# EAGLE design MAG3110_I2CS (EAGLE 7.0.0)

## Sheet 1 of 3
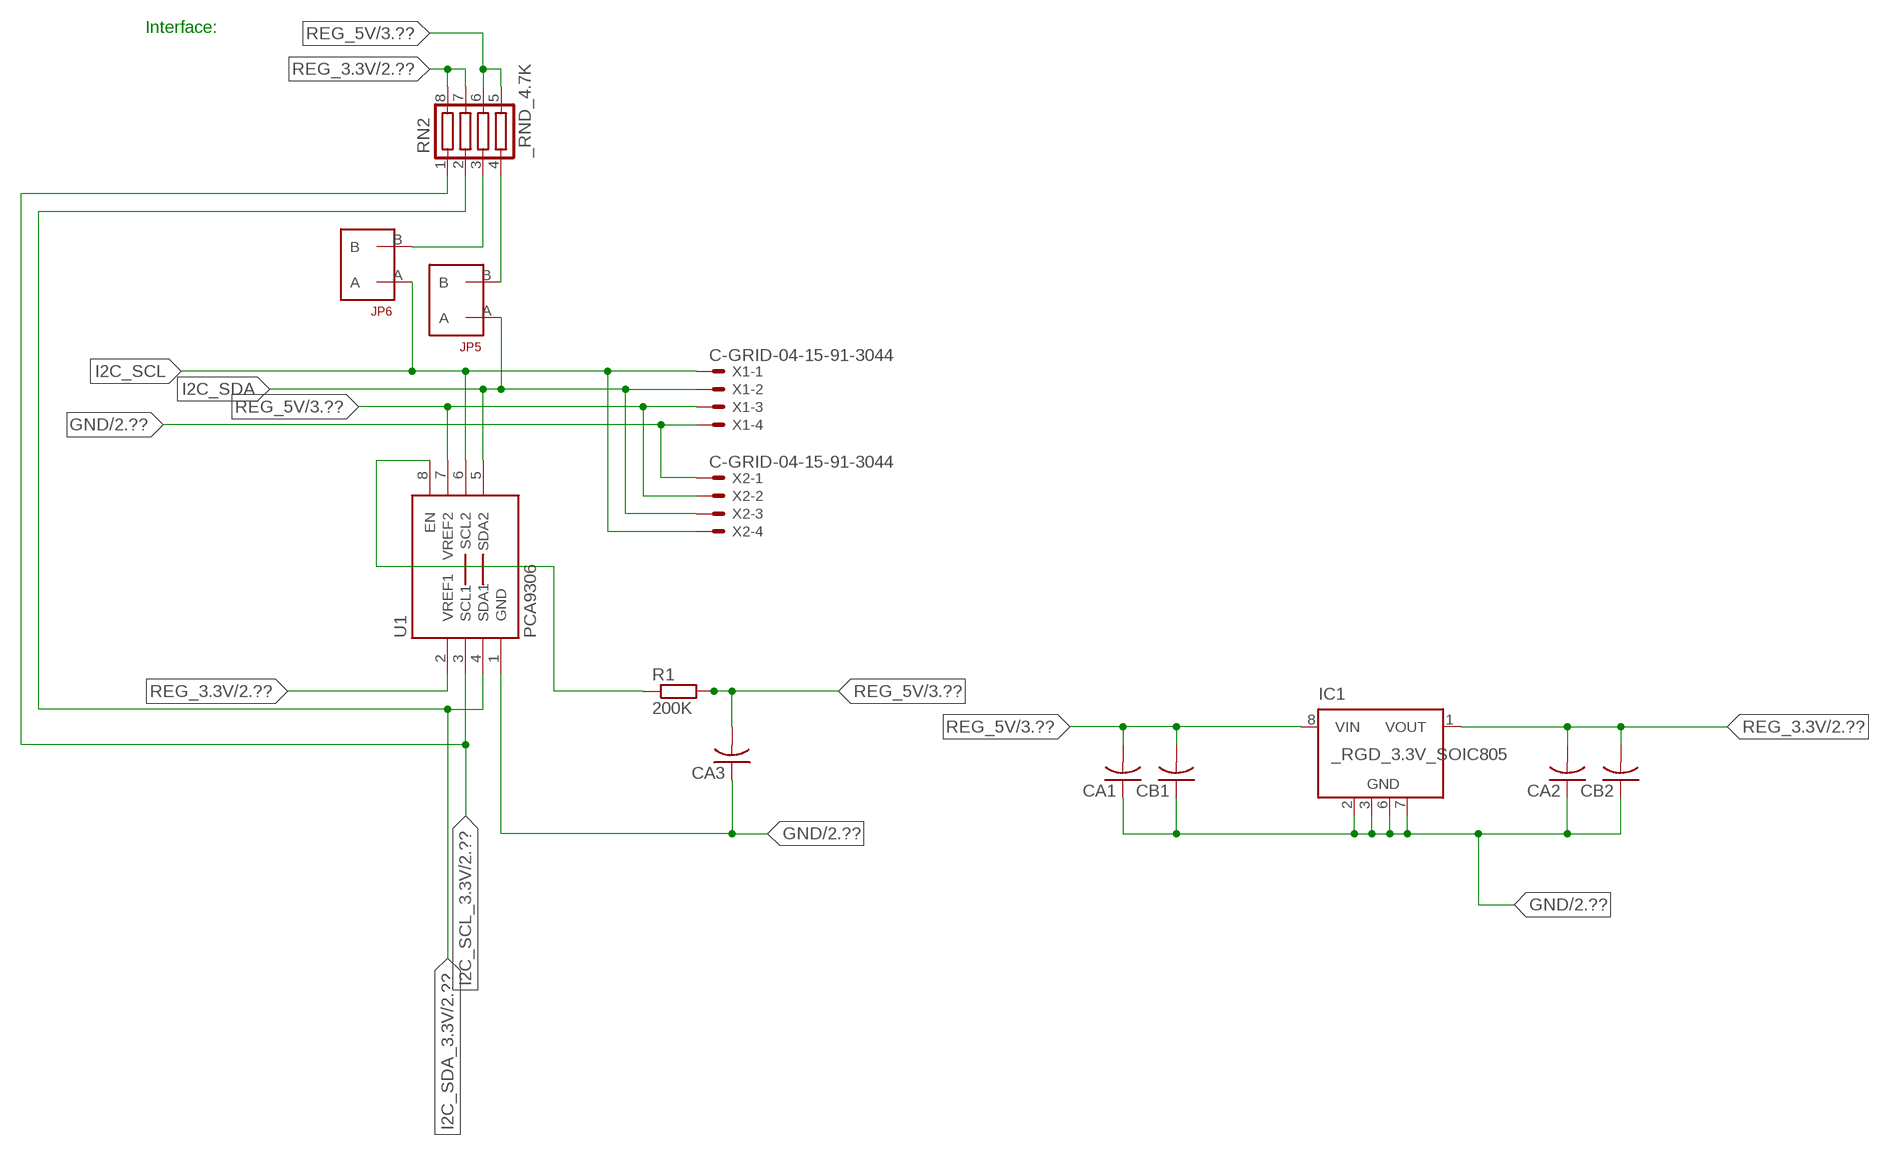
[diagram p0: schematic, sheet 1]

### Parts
CA1  CC1206KRX7R9BB104  [.1UF]
CA2  CC1206KRX7R9BB104  [.1UF]
CA3  CC1206KRX7R9BB104  [.1UF]
CB1  TMK316F106ZL-TC1206K  [TMK316F106ZL-T]
CB2  TMK316F106ZL-TC1206K  [TMK316F106ZL-T]
IC1  _RGD_3.3V_SOIC805  [_RGC_3.3V_SOIC8]
JP5  JUMPER_1X2_2MM  [JUMPER_1X2_2MM]
JP6  JUMPER_1X2_2MM  [JUMPER_1X2_2MM]
R1  200K  RESISTOR_SMT-0603  [R603]
RN2  _RND_4.7K  [RND]
U1  PCA9306  PCA9306_NCD  [PSOP-8]
X1  C-GRID-04-15-91-3044  [15-91-04]
X2  C-GRID-04-15-91-3044  [15-91-04]

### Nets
GND: CA1.1 CA2.1 CA3.1 CB1.1 CB2.1 IC1.2(GND) IC1.3(GND) IC1.6(GND) IC1.7(GND) U1.1(GND) X1.4 X2.1 ; also sheet 2,3
I2C_SCL: JP6.A U1.6(SCL2) X1.1 X2.4
I2C_SCL_3.3V: RN2.1 U1.3(SCL1) ; also sheet 2
I2C_SDA: JP5.A U1.5(SDA2) X1.2 X2.3
I2C_SDA_3.3V: RN2.2 U1.4(SDA1) ; also sheet 2
N$1: JP6.B RN2.3
N$2: JP5.B RN2.4
N$3: R1.1 U1.8(EN)
REG_3.3V: CA2.2 CB2.2 IC1.1(VOUT) RN2.7 RN2.8 U1.2(VREF1) ; also sheet 2
REG_5V: CA1.2 CA3.2 CB1.2 IC1.8(VIN) R1.2 RN2.5 RN2.6 U1.7(VREF2) X1.3 X2.2 ; also sheet 3
Unconnected: IC1.4(NC) IC1.5(NC)

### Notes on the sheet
- Interface:

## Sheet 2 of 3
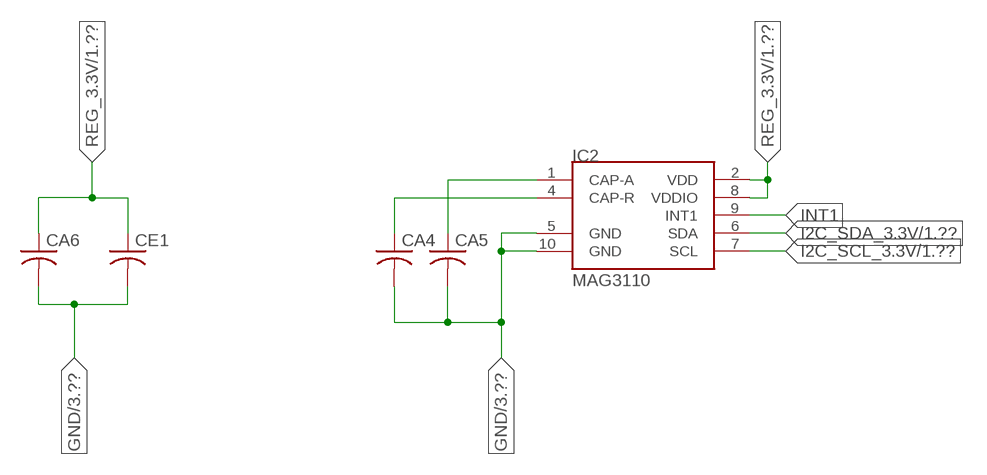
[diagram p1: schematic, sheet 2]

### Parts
CA4  CC1206KRX7R9BB104  [.1UF]
CA5  CC1206KRX7R9BB104  [.1UF]
CA6  CC1206KRX7R9BB104  [.1UF]
CE1  CC0603JRNPO8BN1020603  [CC0603JRNPO8BN102]
IC2  MAG3110  [DFN-10]

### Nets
GND: CA4.2 CA5.2 CA6.2 CE1.2 IC2.5(GND) IC2.10(GND) ; also sheet 1,3
I2C_SCL_3.3V: IC2.7(SCL) ; also sheet 1
I2C_SDA_3.3V: IC2.6(SDA) ; also sheet 1
INT1: IC2.9(INT1)
N$5: CA5.1 IC2.1(CAP-A)
N$6: CA4.1 IC2.4(CAP-R)
REG_3.3V: CA6.1 CE1.1 IC2.2(VDD) IC2.8(VDDIO) ; also sheet 1

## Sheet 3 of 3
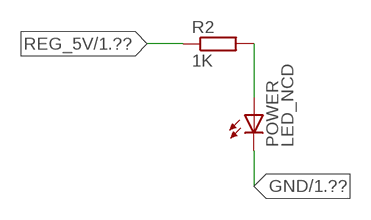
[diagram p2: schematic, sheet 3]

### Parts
POWER  LED_NCD  [CHIPLED_0603]
R2  1K  RESISTOR_SMT-0402  [R402]

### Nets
GND: POWER.C ; also sheet 1,2
N$4: POWER.A R2.2
REG_5V: R2.1 ; also sheet 1

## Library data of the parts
CA1-CA6 = NCD_ULTIMATE_LIBRARY:CC1206KRX7R9BB104: Capacitor CA .1uF 50V SMT C1206K CC1206KRX7R9BB104
CB1 CB2 = NCD_ULTIMATE_LIBRARY:TMK316F106ZL-T: Capacitor CB 10uF SMT 1206 TMK316F106ZL-T
CE1 = NCD_ULTIMATE_LIBRARY:CC0603JRNPO8BN102: Capacitor CE 1uF SMT CC0603JRNPO8BN102 0603
IC1 = NCD_ULTIMATE_LIBRARY:_RGD_3.3V_SOIC8: Regulator Linear 3.3V Chip Positive VOLTAGE REGULATOR Digikey 497-1199-2-ND/L78L33ACD13TR
IC2 = SparkFun-Sensors:MAG3110: 3-axis digital (I2C) magnetometer
JP5 JP6 = NCD_ULTIMATE_CONNECTORS:JUMPER_1X2_2MM
POWER = NCD_ULTIMATE_LIBRARY:LED_NCD: LED Digikey 754-1132-2-ND/APT2012SRCPRV
R1 R2 = NCD_ULTIMATE_LIBRARY:RESISTOR_SMT: NCD Resistor
RN2 = NCD_ULTIMATE_LIBRARY:_RND_4.7K: Resistor Array RND SMT 4.7K x 4 Single Resistor Source: http://www.ctscorp.com/components/Datasheets/CTSChipArrayDs.pdf Digikey 742C083472JPTR-ND/742C083472JP; OC_FARNELL: unknown; OC_NEWARK: unknown
U1 = NCD_ULTIMATE_LIBRARY:PCA9306_NCD: NCD Bidirectional I2C level shifter. NOT compatible with all available part number pinout schemes- DOUBLE CHECK!!!; PROD_ID: IC-10023
X1 X2 = NCD_ULTIMATE_CONNECTORS:C-GRID-04: CONNECTOR 4-Pos I2C wire to board 2.54 mm (0.100") pitch header Digikey WM1342-ND/0015912045; OC_FARNELL: unknown; OC_NEWARK: unknown

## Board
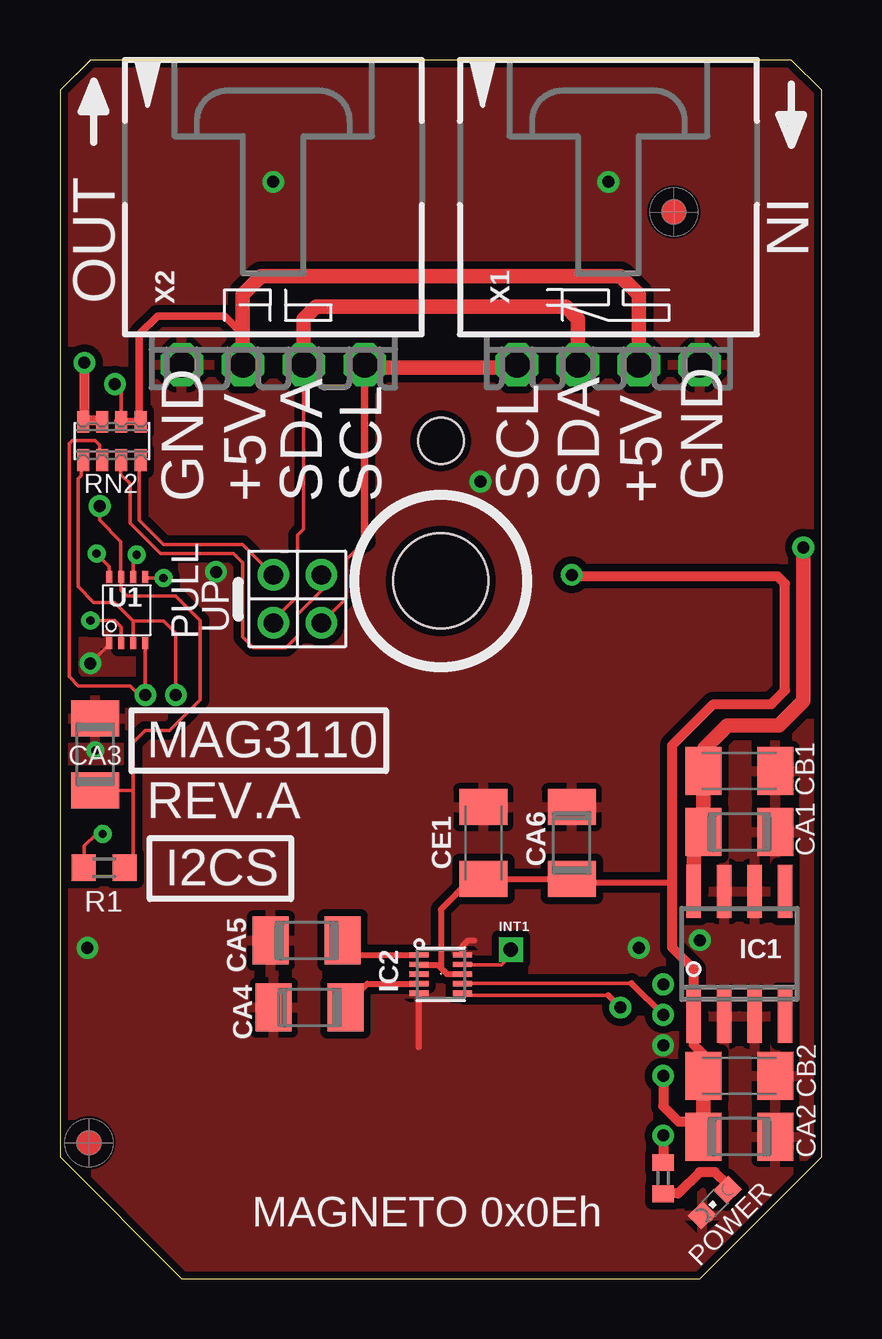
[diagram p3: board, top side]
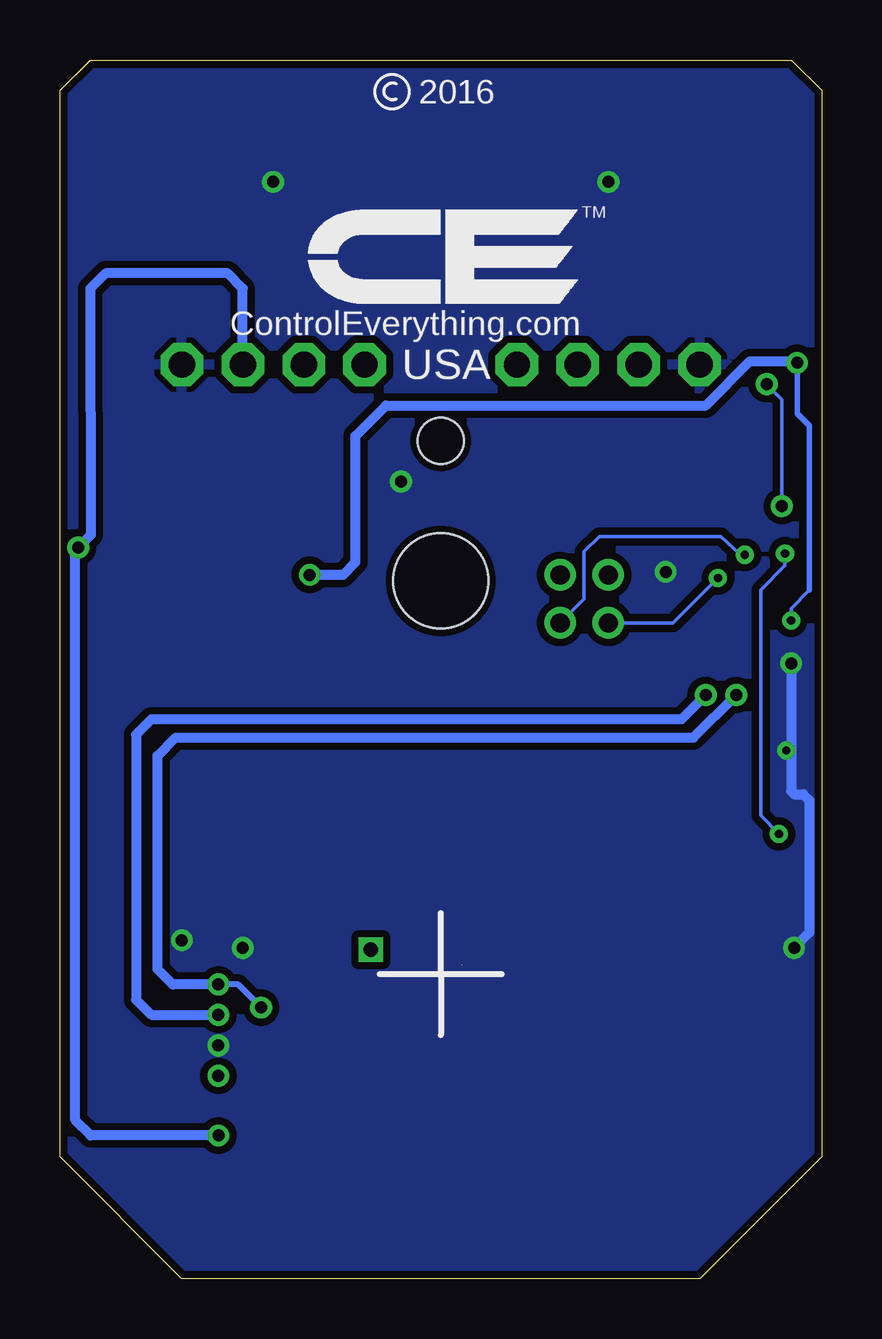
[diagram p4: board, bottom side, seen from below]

Size 31.75 x 50.8 mm. Coordinates in mm from the lower left corner, seen from the top.
Outline: 32 segments
Copper layers (1*16): Top 0.035mm / dielectric 1.5mm / Bottom 0.035mm
Design rules "default": minimum track width 5mil, minimum drill 24mil, track to track 5mil, track to pad 5mil, pad to pad 5mil, via to via 5mil, smd to smd 5mil, copper to edge 10mil, drill to drill 8mil, minimum pad ring 10mil, minimum via ring 8mil, stop-mask expansion 2mil, vias tented up to drill 0mil, thermal gap 10mil
Holes 3.96 mm at 15.88,29.08
Holes 1.91 mm at 15.88,34.93

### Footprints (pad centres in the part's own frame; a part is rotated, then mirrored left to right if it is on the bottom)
.1UF = smd 1.5 x 2: 1 -1.5,0; 2 1.5,0
TMK316F106ZL-T = smd 1.5 x 2: 1 -1.5,0; 2 1.5,0
CC0603JRNPO8BN102 = smd 1.5 x 2: 1 -1.5,0; 2 1.5,0
_RGC_3.3V_SOIC8 = smd 0.6 x 2.2: 1 -1.905,-2.6; 2 -0.635,-2.6; 3 0.635,-2.6; 4 1.905,-2.6; 5 1.905,2.6; 6 0.635,2.6; 7 -0.635,2.6; 8 -1.905,2.6
DFN-10 = smd 0.8 x 0.22: 1 -0.91,0.8; 2 -0.91,0.4; 3 -0.91,0; 4 -0.91,-0.4; 5 -0.91,-0.8; 6 0.91,-0.8; 7 0.91,-0.4; 8 0.91,0; 9 0.91,0.4; 10 0.91,0.8
JUMPER_1X2_2MM = drill 0.8: A 0,2; B 0,0
CHIPLED_0603 = smd 0.8 x 0.876: A 0,-0.75; C 0,0.75
R603 = smd 1 x 1.1: 1 -0.85,0; 2 0.85,0
R402 = smd 0.7 x 0.9: 1 -0.65,0; 2 0.65,0
RND = smd 0.5 x 0.9: 1 -1.2,-0.8; 2 -0.4,-0.8; 3 0.4,-0.8; 4 1.2,-0.8; 5 1.2,0.8; 6 0.4,0.8; 7 -0.4,0.8; 8 -1.2,0.8
PSOP-8 = smd 0.25 x 0.5: 1 -0.73,-1.37; 2 -0.23,-1.37; 3 0.27,-1.37; 4 0.77,-1.37; 5 0.77,1.38; 6 0.27,1.38; 7 -0.23,1.38; 8 -0.73,1.38
15-91-04 = drill 1.1 pad 1.778 octagon: 1 -3.81,-7.62; 2 -1.27,-7.62; 3 1.27,-7.62; 4 3.81,-7.62

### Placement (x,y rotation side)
CA1  28.32,18.62 180 top
CA2  28.32,5.92 180 top
CA3  1.46,21.86 270 top
CA4  10.41,11.3 180 top
CA5  10.29,14.1 180 top
CA6  21.34,18.16 90 top
CB1  28.32,21.16 180 top
CB2  28.32,8.46 180 top
CE1  17.65,18.16 90 top
IC1  28.32,13.54 0 top
IC2  15.88,12.7 0 top
JP5  8.89,29.34 180 top
JP6  10.9,29.34 180 top
POWER  27.3,3.18 135 top
R1  1.84,17.13 0 top
R2  25.15,4.19 270 top
RN2  2.16,34.93 0 top
U1  2.79,27.86 0 top
U$5  [VISION_REF10]  1.21,5.66 90 top
U$28  [VISION_REF10]  25.59,44.46 90 top
X1  22.86,45.72 0 top
X2  8.89,45.72 0 top

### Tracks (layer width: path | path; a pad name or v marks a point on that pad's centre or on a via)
GND  (via drill 0.35, 0.5)
  Top 0.152: CA3.1 1.52,23.42 1.52,23.62 | v1.27,25.65 2.06,26.45 U1.1
  Top 0.254: 14.96,9.65 IC2.5 | IC2.10 16.79,13.86 17.02,14.1 17.27,14.1
  Bottom 0.152: 1.27,20.32 1.14,20.19
  Bottom 0.406: v1.15,13.79 0.51,14.43 0.51,19.94 0.76,20.19 1.14,20.19 | v1.27,25.65 1.27,20.32
  other vias: 8.89,45.72 22.86,45.72 25.15,9.73 17.53,33.22 26.67,14.11 6.5,29.46 1.47,22.02 24.13,13.79
  pour Bottom (isolate 0.305): -0.64,5.08 -0.64,49.53 1.27,51.44 30.48,51.44 32.38,49.53 32.38,5.08 26.67,-0.63 5.08,-0.63
  pour Top (isolate 0.305): 4.45,-1.27 -1.27,4.45 -1.27,50.17 0.64,52.07 31.11,52.07 33.02,50.17 33.02,4.45 27.3,-1.27
I2C_SCL  (via drill 0.35)
  Top 0.152: 12.7,30.73 11.94,29.97 11.94,28.38 JP6.A | v3.2,30.18 3.06,29.99 U1.6
  Top 0.305: 12.7,30.73 X2.4
  Top 0.406: X2.4 12.7,37.97 | 19.05,37.97 X1.1
  Top 0.61: 12.7,37.97 19.05,37.97
  Bottom 0.152: JP6.A 9.91,28.33 9.91,30.3 9.27,30.94 4.19,30.94 3.38,30.18 v3.2,30.18
I2C_SCL_3.3V  (via drill 0.5)
  Top 0.152: RN2.1 0.89,34.07 0.89,33.48 0.77,33.35 0.77,28.84 1.41,28.19 2.29,28.19 3.06,27.42 | 23.83,12.32 16.8,12.32 IC2.7 | 3.06,27.42 U1.3 | v4.83,24.33 v4.83,24.34 4.83,26.92 4.33,27.42 3.06,27.42
  Top 0.254: 23.83,12.32 v25.15,11
  Bottom 0.406: v4.83,24.33 5.84,23.32 27.94,23.32 28.58,22.68 28.58,11.63 27.94,11 v25.15,11
I2C_SDA  (via drill 0.35)
  Top 0.152: JP5.A 8.89,27.44 9.91,28.45 9.91,30.99 10.16,31.24 10.16,34.92 X2.3 | U1.5 3.6,29.21 v4.32,29.21
  Top 0.61: X2.3 10.16,40.01 10.67,40.51 21.09,40.51 21.59,40.01 X1.2
  Bottom 0.152: v4.32,29.21 6.19,27.34 JP5.A
I2C_SDA_3.3V  (via drill 0.5)
  Top 0.152: RN2.2 1.65,34.14 1.65,34.75 1.46,34.94 0.51,34.94 0.38,34.81 0.38,26.37 0.38,26.36 0.38,25.1 0.76,24.71 2.92,24.71 3.3,24.33 v3.56,24.33 U1.4 | 22.86,11.81 16.87,11.81 IC2.6
  Top 0.254: 22.86,11.81 v23.37,11.3
  Bottom 0.254: v23.37,11.3 24.33,12.27 v25.15,12.27
  Bottom 0.406: v25.15,12.27 27.05,12.27 27.69,12.9 27.69,21.79 26.93,22.56 5.34,22.56 v3.56,24.33
INT1  (via drill 0.6)
  Top 0.152: 18.8,13.46 18.41,13.08 16.8,13.08 IC2.9
  Top 0.254: 18.8,13.46 v18.8,13.72
N$1
  Top 0.152: JP6.B 10.92,29.31 10.92,28.7 9.91,27.69 9.91,26.8 9.42,26.31 8.06,26.31 7.62,26.75 7.62,29.84 7.24,30.23 4.19,30.23 2.92,31.5 2.92,33.15 2.54,33.53 2.54,34.1 RN2.3
  Top 0.305: 2.54,34.02 RN2.3
N$2
  Top 0.152: JP5.B 7.62,30.61 4.32,30.61 3.3,31.62 3.3,34.07 RN2.4
  Top 0.305: 3.37,33.88 RN2.4
N$3  (via drill 0.35)
  Top 0.152: R1.1 1.02,17.16 1.02,18.03 1.52,18.54 v1.78,18.54 | v1.52,30.23 2.06,29.69 U1.8
  Bottom 0.152: v1.78,18.54 2.54,19.3 2.54,28.7 1.52,29.72 v1.52,30.23
N$4
  Top 0.406: POWER.A 27.84,3.92 27.3,4.45 26.67,4.45 25.78,3.56 25.16,3.56 R2.2
N$5
  Top 0.254: CA5.1 12.38,13.5 IC2.1
N$6
  Top 0.254: CA4.1 11.91,11.41 12.81,12.3 IC2.4
REG_3.3V  (via drill 0.35, 0.5)  (1 unrouted)
  Top 0.152: v1.27,27.43 2.29,27.43 2.56,27.16 U1.2
  Top 0.254: 14.98,13.08 15.75,13.08 15.88,12.95 | 15.88,12.95 16.13,12.7 IC2.8 | 15.88,12.95 15.88,15.39 17.14,16.66 CE1.1 CA6.1 21.49,16.51 25.53,16.51 | 25.15,7.88 v25.15,8.46
  Top 0.406: CB2.2 26.82,9.35 26.42,9.75 26.42,10.36 | v25.15,8.46 25.15,7.19 25.78,6.55 26.82,6.55 | IC1.1 26.42,12.9 25.53,13.79 25.53,16.51 25.53,22.24 27.24,23.95 29.66,23.95 30.23,24.52 30.23,28.97 29.91,29.29 21.39,29.29 v21.34,29.34 | 26.52,5.62 CA2.2 | v1.02,38.18 1.02,35.78 | 1.02,35.78 RN2.8 | 1.02,35.78 1.71,35.78 RN2.7
  Top 0.61: CB2.2 26.82,6.55 CA2.2 | 26.42,10.36 IC1.1
  Bottom 0.152: 0.51,28.7 1.27,27.94 v1.27,27.43
  Bottom 0.229: 0.51,28.7 0.51,35.56 1.02,36.07 v1.02,38.18
  Bottom 0.406: v1.02,38.18 1.08,38.24 2.99,38.24 4.83,36.4 18.16,36.4 19.43,35.13 19.43,29.87 19.94,29.34 v21.34,29.34
REG_5V  (via drill 0.5)
  Top 0.152: RN2.6 2.56,37.01 v2.29,37.29 | R1.2 3.05,17.49 3.05,20.36 | 3.05,20.36 3.05,22.35 3.56,22.86 4.57,22.86 5.84,24.13 5.84,27.43 4.83,28.45 2.79,28.45 2.56,28.68 U1.7 2.54,29.27 2.54,30.73 1.65,31.62 v1.65,32.21 | CA3.2 3.05,20.36
  Top 0.305: 7.62,39.37 7.5,39.37 | 2.42,35.74 RN2.6 RN2.5 3.31,35.8 3.31,39.37 4.07,40.13 6.86,40.13 7.62,39.37 | X2.2 7.62,39.37
  Top 0.406: v25.15,5.97 R2.1
  Top 0.61: X1.3 24.13,41.02 23.37,41.78 8.38,41.78 7.62,41.02 X2.2 | IC1.8 26.42,18.21 CA1.2 CB1.2 26.86,21.2 26.86,22.11 27.82,23.06 29.98,23.06 30.99,24.08 v30.99,30.48
  Bottom 0.152: v1.65,32.21 1.65,36.65 v2.29,37.29
  Bottom 0.406: X1.3 24.13,41.28 24.77,41.91 29.84,41.91 30.48,41.27 30.47,31 v30.99,30.48 31.11,30.36 31.11,6.6 30.48,5.97 v25.15,5.97

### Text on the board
tNames: IN | OUT | GND | +5V | SDA | SCL | SCL | SDA | +5V | GND | PULL | UP | MAG3110 | REV.A | I2CS | INT1 | MAGNETO 0x0Eh
bNames: 2016 | TM | ControlEverything.com | USA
